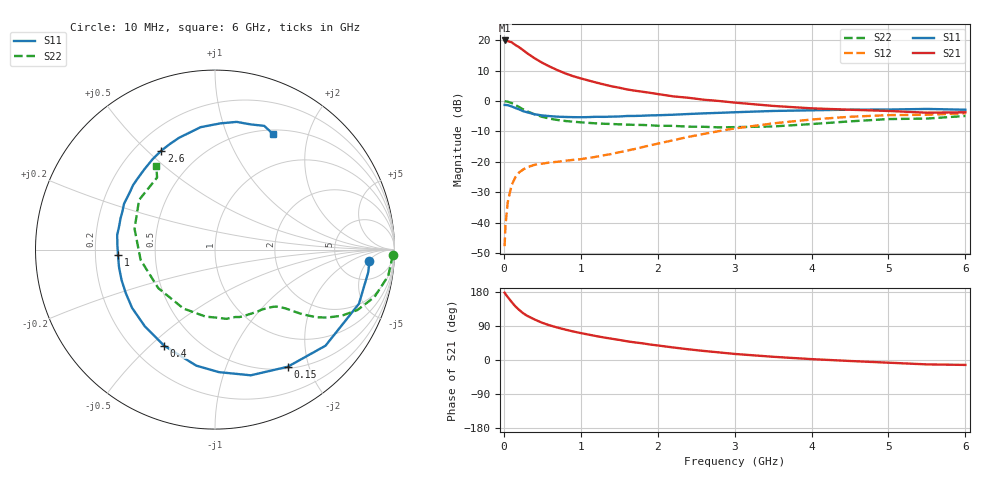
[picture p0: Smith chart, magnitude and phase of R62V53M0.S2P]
! SIEMENS Small Signal Semiconductors
! BFR193
! Si NPN RF Bipolar Junction Transistor in SOT23
! VCE = 2.5 V  IC = 3 mA
! Common Emitter S-Parameters:  May  1996
# GHz  S  MA  R  50
!  f  S11  S21  S12  S22
! GHz  MAG  ANG  MAG  ANG  MAG  ANG  MAG  ANG
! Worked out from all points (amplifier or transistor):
!   36 points, 10 MHz to 6 GHz, reference 50 ohm
!   highest |S21| = 19.9 dB at 10 MHz (marker M1)
!   |S21| within 3 dB of that: start of sweep to 240.6 MHz
!   unconditionally stable (mu >= 1): 1.031 GHz to 2.051 GHz
!   at 250 MHz: K = 0.31, MSG = 19.7 dB, |S12| = -22.5 dB
!   at 1.4 GHz: K = 1.10, MAG = 9.2 dB, |S12| = -17.4 dB
!   at 6 GHz: K = 0.98, MSG = 0.2 dB, |S12| = -4.0 dB
!   S11 on the Smith chart (normalised r, x): 10 MHz: 11, -5; 150 MHz: 0.53, -1.67; 400 MHz: 0.33, -0.55; 1 GHz: 0.30, -0.02; 2.6 GHz: 0.30, +0.55; 6 GHz: 0.56, +1.48
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0.01  0.863 -4.3  9.926 177.5  0.0041 89.1  0.9948 -1.8
0.02  0.8629 -8.5  9.785 174.4  0.0086 81.9  0.9862 -3.5
0.05  0.8569 -20.6  9.689 166.3  0.0215 78.2  0.9759 -8.7
0.1  0.816 -41.0  9.289 153.4  0.0411 69.3  0.9264 -16.6
0.15  0.7682 -58.2  8.361 141.5  0.0558 60.9  0.862 -23.0
0.2  0.7282 -74.1  7.657 132.0  0.0671 54.7  0.7959 -27.6
0.25  0.683 -88.2  6.889 123.6  0.0746 49.7  0.7306 -31.2
0.3  0.6548 -99.2  6.154 117.0  0.0812 46.2  0.68 -33.7
0.4  0.6055 -118.0  5.056 106.9  0.0894 41.5  0.6055 -36.5
0.5  0.5794 -132.4  4.256 98.1  0.0936 39.4  0.5495 -38.4
0.6  0.5648 -144.9  3.673 91.2  0.0976 39.1  0.5121 -39.8
0.8  0.5475 -162.0  2.846 80.2  0.1041 40.7  0.4697 -42.6
1  0.5415 -176.9  2.357 71.0  0.1107 44.5  0.4469 -45.9
1.1  0.5447 177.1  2.179 67.1  0.1157 46.9  0.4376 -48.1
1.3  0.5495 166.8  1.875 59.5  0.1281 51.3  0.4229 -52.5
1.6  0.5677 153.2  1.554 49.4  0.1529 56.5  0.4096 -60.6
2.2  0.5956 131.5  1.195 33.1  0.2264 59.8  0.3908 -80.7
2.6  0.6275 118.4  1.052 23.9  0.2881 57.0  0.3772 -97.9
3.5  0.6868 96.7  0.832 8.5  0.4291 43.0  0.382 -145.8
4.5  0.7217 80.4  0.72 -2.6  0.5513 24.0  0.463 165.5
5.5  0.7419 68.3  0.643 -11.6  0.5949 5.7  0.5151 128.8
6  0.7198 63.1  0.654 -13.0  0.6302 0.6  0.5682 125.1
